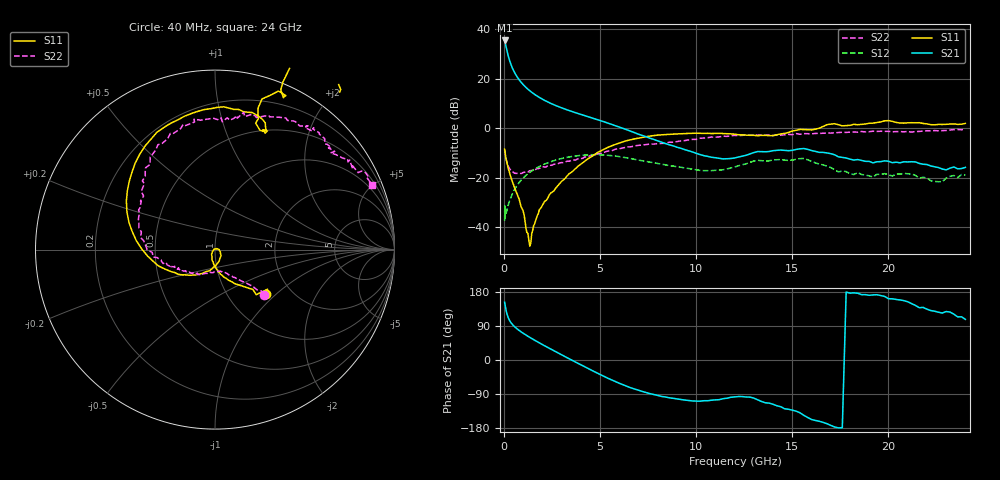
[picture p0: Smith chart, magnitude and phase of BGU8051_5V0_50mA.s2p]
! BGU8051_5V0_50mA
! Date/time Tue Jun 16 11:08:37 2015
! VAR V_out= 5.0010
! VAR I_out= 50.0000
! VAR V_in= 5.4890
! VAR I_in= 0.6779
# MHz S MA R 50
!  Freq-MHz  S11-mag  S11-arg  S21-mag  S21-arg  S12-mag  S12-arg  S22-mag  S22-arg
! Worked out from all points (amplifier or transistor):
!   187 points, 40 MHz to 24 GHz, reference 50 ohm
!   highest |S21| = 35.6 dB at 40 MHz (marker M1)
!   |S21| within 3 dB of that: start of sweep to 127.5 MHz
!   unconditionally stable (mu >= 1): 401.7 MHz to 14.04 GHz
!   at 750 MHz: K = 1.02, MAG = 20.4 dB, |S12| = -22.4 dB
!   at 5.4 GHz: K = 1.19, MAG = 3.9 dB, |S12| = -10.9 dB
!   at 24 GHz: K = -1.05, MSG = 1.6 dB, |S12| = -18.9 dB
!   lowest NFmin = 0.38 dB at 400 MHz
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40  0.3789 -41.3  59.92 152.6  0.01357 36.5  0.3711 -42.5
60  0.3403 -47.5  55.74 146.8  0.01959 20.2  0.3259 -43.7
80  0.2922 -48.1  51.12 141.0  0.01675 38.6  0.2784 -45.2
120  0.2396 -55.7  43.68 130.4  0.01962 45.3  0.2341 -49.3
160  0.2016 -62.6  37.26 122.1  0.02185 50.0  0.2053 -52.9
200  0.1729 -68.6  32.14 115.7  0.02506 55.0  0.1839 -56.5
260  0.1408 -77.4  26.42 108.1  0.03074 57.9  0.1619 -60.5
320  0.1156 -82.6  22.25 102.5  0.03599 59.8  0.1476 -63.8
400  0.09234 -90.5  18.27 96.6  0.04358 61.7  0.137 -67.7
500  0.07315 -96.9  14.9 90.8  0.05272 62.4  0.1288 -73.5
700  0.04571 -111.2  10.86 81.7  0.07125 60.8  0.1227 -81.5
900  0.02567 -129.9  8.532 74.2  0.08939 57.9  0.1219 -90.6
1350  0.004125 114.9  5.738 59.7  0.1291 49.9  0.1388 -105.8
1500  0.008534 35.4  5.176 55.2  0.1417 46.9  0.1408 -110.5
2500  0.05039 -50.1  3.116 27.2  0.2152 25.4  0.1795 -133.4
4100  0.1999 -134.3  1.861 -15.1  0.2859 -10.4  0.2471 -157.2
5600  0.4415 173.5  1.202 -52.4  0.2795 -42.8  0.35 -177.4
8200  0.7388 112.3  0.5244 -96.2  0.188 -76.2  0.4954 147.0
12200  0.743 67.8  0.2626 -96.4  0.1746 -75.8  0.7103 103.4
16200  0.9625 67.6  0.3414 -159.5  0.2001 -149.1  0.7882 70.3
20200  1.383 34.6  0.2016 161.5  0.1086 -159.6  0.8498 43.9
24000  1.255 21.9  0.1622 107.3  0.1134 -179.6  0.9478 22.2
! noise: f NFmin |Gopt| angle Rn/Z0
400  0.3819  0.06119  79.21  0.0479
550  0.3881  0.05606  98.18  0.048
950  0.4174  0.0686  142.4  0.0483
1250  0.4516  0.08966  160.3  0.0487
1600  0.5048  0.1158  172.4  0.0495
1900  0.5617  0.1374  179.5  0.0507
2250  0.6415  0.1611  186.1  0.0531
2600  0.7355  0.1834  191.6  0.0567
3300  0.9663  0.2269  201.3  0.0689
4000  1.254  0.2736  209.9  0.0897
